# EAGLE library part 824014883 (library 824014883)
ESD Suppressors / TVS Diodes WE-TVS Diode Array 3.3V 0.5pF 8Channel Source: Datasheet
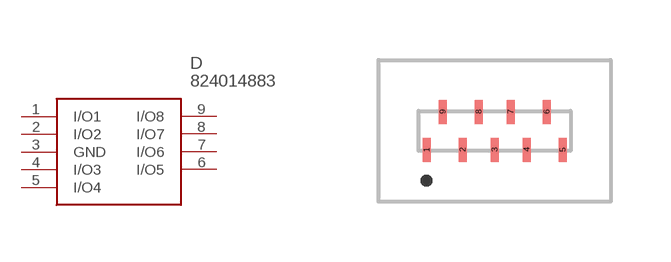
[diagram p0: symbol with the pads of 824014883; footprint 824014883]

Designator prefix D

## 824014883 (Description: ESD Suppressors / TVS Diodes WE-TVS Diode Array 3.3V 0.5pF 8Channel; Height: 0.55mm; Manufacturer_Name: Wurth Elektronik; Manufacturer_Part_Number: 824014883; Mouser_Part_Number: 710-824014883; Mouser_Price-Stock: https://www.mouser.co.uk/ProductDetail/Wurth-Elektronik/824014883?qs=rrS6PyfT74cNUdMCm8eE6Q%3D%3D)  [824014883]
1  I/O1
2  I/O2
3  GND
4  I/O3
5  I/O4
6  I/O5
7  I/O6
8  I/O7
9  I/O8

## Footprint 824014883 (pad centres in mm)
824014883-2
smd 0.2 x 0.6: 1 -1.7,-0.475; 2 -0.8,-0.475; 3 0,-0.475; 4 0.8,-0.475; 5 1.7,-0.475; 6 1.3,0.475; 7 0.4,0.475; 8 -0.4,0.475; 9 -1.3,0.475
